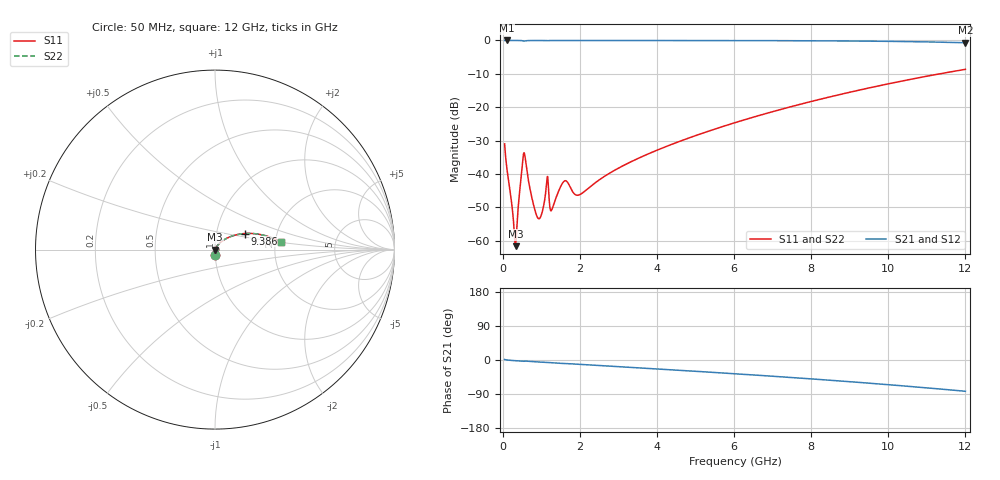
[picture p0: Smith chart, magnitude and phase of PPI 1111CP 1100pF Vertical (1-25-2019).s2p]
# GHz S MA R 50
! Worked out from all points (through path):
!   1601 points, 50 MHz to 12 GHz, reference 50 ohm
!   highest |S21| = 0.00 dB at 109.8 MHz (marker M1); lowest = -0.7 dB at 12 GHz (marker M2)
!   group delay of S21, straight-line fit = 18.8 ps
!   lowest |S11| = -61.7 dB at 333.8 MHz (marker M3), VSWR 1.00, Z = 50.1 + j0.00126 ohm
!   |S11| at or under -10 dB: start of sweep to 11.34 GHz
!   |S22| runs from -61.7 to -8.7 dB; largest |S21 - S12| = 0
!   S11 on the Smith chart (normalised r, x): 50 MHz: 1.00, -0.06; 9.386 GHz: 1.37, +0.25; 12 GHz: 2.14, +0.21
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0.05  0.02817 -88.0  0.9993 1.3  0.9993 1.3  0.02817 -88.0
0.10975  0.01198 -88.0  0.9995 0.1  0.9995 0.1  0.01198 -88.0
0.289  0.001676 -67.6  0.9993 -1.5  0.9993 -1.5  0.001676 -67.6
0.3338125  0.0008247 0.9  0.9992 -1.9  0.9992 -1.9  0.0008247 0.9
0.378625  0.00208 55.9  0.9989 -2.2  0.9989 -2.2  0.00208 55.9
0.498125  0.01195 51.1  0.993 -3.4  0.993 -3.4  0.01195 51.1
0.557875  0.02066 -2.5  0.9793 -3.2  0.9793 -3.2  0.02066 -2.5
0.7894062  0.003648 -47.4  0.9973 -4.3  0.9973 -4.3  0.003648 -47.4
0.9238437  0.002143 -8.3  0.9978 -5.2  0.9978 -5.2  0.002143 -8.3
1.020938  0.002619 29.1  0.9978 -5.9  0.9978 -5.9  0.002619 29.1
1.140437  0.007415 36.4  0.9945 -6.7  0.9945 -6.7  0.007415 36.4
1.274875  0.002902 23.0  0.9974 -7.3  0.9974 -7.3  0.002902 23.0
1.6035  0.007837 29.9  0.9938 -9.3  0.9938 -9.3  0.007837 29.9
1.879844  0.004899 21.6  0.9957 -10.7  0.9957 -10.7  0.004899 21.6
2.044156  0.005053 40.1  0.9967 -11.7  0.9967 -11.7  0.005053 40.1
2.873187  0.01107 61.0  0.9974 -16.7  0.9974 -16.7  0.01107 61.0
4.038312  0.02309 60.0  0.997 -23.8  0.997 -23.8  0.02309 60.0
6.025  0.05857 50.8  0.995 -36.3  0.995 -36.3  0.05857 50.8
8.019156  0.1224 38.3  0.9884 -50.0  0.9884 -50.0  0.1224 38.3
9.385938  0.1878 28.5  0.9774 -60.2  0.9774 -60.2  0.1878 28.5
10.01331  0.2245 23.6  0.9694 -65.2  0.9694 -65.2  0.2245 23.6
12  0.3688 6.6  0.9232 -82.5  0.9232 -82.5  0.3688 6.6
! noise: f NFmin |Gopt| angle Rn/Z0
0.05  0.0003793  0.8684  0.299  0.00062
1.372  0.005846  0.7779  7.74  0.005364
2.701  0.0078  0.6917  15.13  0.004846
4.031  0.009715  0.6469  22.31  0.005031
5.36  0.01179  0.627  29.24  0.005561
6.682  0.01389  0.619  35.81  0.006189
8.012  0.01609  0.6193  42.07  0.00692
9.341  0.01843  0.6261  47.97  0.007783
10.67  0.02097  0.6382  53.53  0.008823
12  0.02379  0.6546  58.76  0.0101
